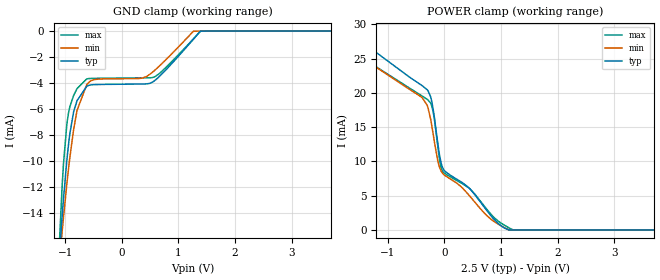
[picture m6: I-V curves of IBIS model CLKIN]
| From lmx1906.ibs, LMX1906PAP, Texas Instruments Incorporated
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|   Model CLKIN
[Model]   CLKIN
Model_type   Input
Vinl = 0.4
Vinh = 1.4
|   typ   min   max
C_comp   0.368pF   0.331pF   0.459pF
[Voltage Range]   2.5   2.4   2.6
[Temperature Range]   27   105   -40
[Power Clamp Reference]   2.5   2.4   2.6
[GND Clamp Reference]   0   0   0
[GND Clamp]
|   Voltage   I(typ)   I(min)   I(max)
-2.5V     -134.6mA   -111.9mA   -211.5mA
-1.127V   -18.74mA   -19.01mA   -18.66mA
-1.052V   -14.15mA   -15.36mA   -11.84mA
-970mV    -9.927mA   -11.74mA   -7.158mA
-917.5mV  -7.895mA   -9.725mA   -5.818mA
-850mV    -6.189mA   -7.55mA    -4.946mA
-790mV    -5.338mA   -6.089mA   -4.414mA
-617.5mV  -4.229mA   -4.1mA     -3.665mA
537.5mV   -3.93mA    -3.173mA   -3.568mA
1.265V    -623.4uA   -12.03uA   -601.9uA
1.385V    -10.48uA   0A         -38.8uA
5V        0A         0A         0A
[POWER Clamp]
|   Voltage   I(typ)   I(min)   I(max)
-2.5V     113.7mA    99.75mA    82.3mA
-1.938V   62.6mA     53.09mA    30.16mA
-1.728V   46.92mA    38.3mA     26.92mA
-1.48V    31.9mA     26.09mA    25.35mA
-1.202V   25.89mA    23.72mA    23.79mA
-302.5mV  20.45mA    18.18mA    19.05mA
-197.5mV  17.68mA    14.06mA    17.27mA
-77.5mV   10.63mA    8.999mA    9.975mA
-17.5mV   8.894mA    8.156mA    8.439mA
447.5mV   6.047mA    4.965mA    6.037mA
1.062V    271uA      327.6uA    696.8uA
5V        0A         0A         0A
